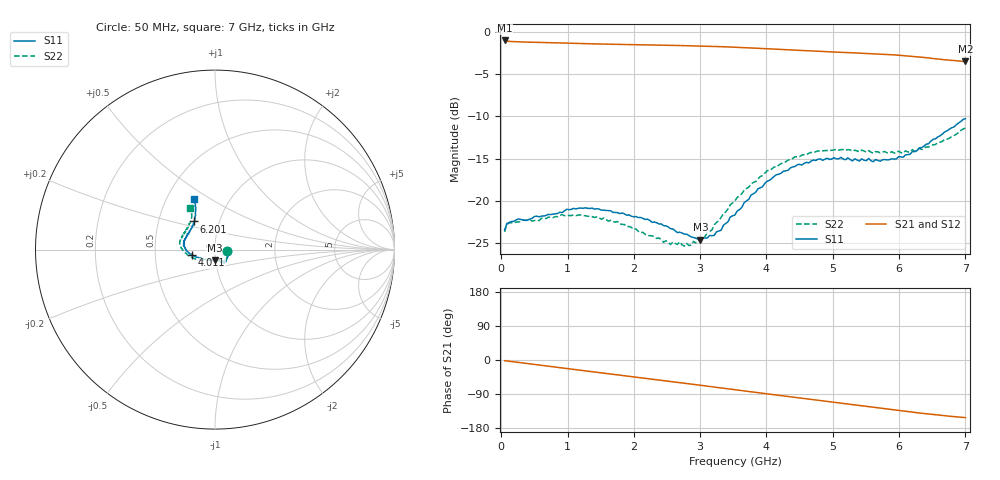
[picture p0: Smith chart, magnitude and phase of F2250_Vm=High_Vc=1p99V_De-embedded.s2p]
! Integrated Device Technology
! Corporate Headquarters
! 6024 Silver Creek Valley Road
! San Jose, CA 95138  USA
! Phone:  1-408-284-8200
! Toll Free:  1-800-223-1366
! Webpage:  http://www.idt.com/
! Timing and RF Division
! 515 Groton Road, Suite 102
! Westford, MA 01886-6024
! Device:  F2250
! Description: Voltage Variable RF Attenuator
! Frequency:  50.0 -  6000.00 MHz
! Package:  3x3 mm Thin QFN Plastic Package: 16 pin
! Ports:  2 RF, 3 DC
!  Pin  1  = GND
!  Pin  2  = NC
!  Pin  3  = RF1  = Port 1
!  Pin  4  = NC
!  Pin  5  = GND
!  Pin  6  = GND
!  Pin  7  = GND
!  Pin  8  = GND
!  Pin  9  = NC
!  Pin 10  = RF2  = Port 2
!  Pin 11  = NC
!  Pin 12  = GND
!  Pin 13  = GND
!  Pin 14  = VCNTRL
!  Pin 15  = VDD
!  Pin 16  = VMODE
! Vcntrl:  1.990 Volts
! Vmode:  +3.300 Volts
! Vdd:  +3.30  Volts
! Current:  1.319 mA
! Data:  The device was measured on a the F2250 evaluation board which has
!  individual transmission lines to the RF pins.  Data was collected
!  using a calibrated network analyzer.  The evaluation board was
!  de-embedded using a TRL calibration technique.
!  The reference plane is the edge of the package pin.
! Misc:  SN 10
!  Action Tracker AT0258
! Date Measured:  2014-11-26
! Date:  2015-10-15  MJV
! Note:
!  Integrated Device Technology supplies this data as a sample of measured
!  data at the package pin for this product.  Your particular data for this
!  product may vary.
!  Data was taken at 25 degrees C.
!  Integrated Device Technology reserves the right to change this data at anytime.
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# GHz S dB R 50
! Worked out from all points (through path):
!   201 points, 50 MHz to 7 GHz, reference 50 ohm
!   highest |S21| = -1.04 dB at 50 MHz (marker M1); lowest = -3.5 dB at 7 GHz (marker M2)
!   group delay of S21, straight-line fit = 61.1 ps
!   lowest |S11| = -24.6 dB at 3.004 GHz (marker M3), VSWR 1.13, Z = 49.5 - j5.88 ohm
!   |S11| at or under -10 dB: start of sweep to end of sweep
!   |S22| runs from -25.3 to -11.4 dB; largest |S21 - S12| = 0.0018
!   S11 on the Smith chart (normalised r, x): 50 MHz: 1.14, -0.02; 4.011 GHz: 0.77, -0.05; 6.201 GHz: 0.76, +0.25; 7 GHz: 0.68, +0.42
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0.05  -23.40 -8.4  -1.04 -1.8  -1.04 -1.8  -23.62 -9.1
0.08475  -22.63 -7.7  -1.12 -2.5  -1.12 -2.5  -22.75 -8.2
0.1195  -22.51 -8.3  -1.15 -3.3  -1.15 -3.3  -22.56 -7.8
0.91875  -21.35 -43.3  -1.34 -21.1  -1.34 -21.1  -21.60 -46.9
1.2315  -20.84 -51.0  -1.41 -27.9  -1.41 -27.9  -21.70 -57.2
1.75275  -21.36 -57.9  -1.50 -39.1  -1.50 -39.1  -22.41 -65.4
2.37825  -22.69 -58.8  -1.59 -52.7  -1.59 -52.7  -24.35 -69.9
2.552  -23.25 -63.0  -1.61 -56.6  -1.61 -56.6  -25.12 -76.5
2.691  -23.67 -69.4  -1.64 -59.7  -1.64 -59.7  -24.81 -83.3
2.7605  -23.89 -71.2  -1.65 -61.2  -1.65 -61.2  -25.32 -87.4
3.00375  -24.55 -91.7  -1.70 -66.7  -1.70 -66.7  -24.37 -108.4
3.21225  -24.03 -113.0  -1.74 -71.4  -1.74 -71.4  -22.80 -126.3
3.525  -21.62 -141.4  -1.84 -78.5  -1.84 -78.5  -19.95 -145.1
3.76825  -19.27 -156.5  -1.93 -84.0  -1.93 -84.0  -17.97 -156.7
4.0115  -17.64 -166.2  -2.03 -89.4  -2.03 -89.4  -16.41 -166.5
4.4285  -15.92 -178.6  -2.19 -98.6  -2.19 -98.6  -14.77 -179.3
4.7065  -15.15 173.9  -2.29 -104.8  -2.29 -104.8  -14.29 174.7
5.054  -15.01 165.6  -2.42 -112.4  -2.41 -112.5  -13.91 167.3
5.85325  -15.11 139.1  -2.71 -129.9  -2.71 -130.0  -14.31 148.2
6.20075  -14.15 126.8  -2.92 -137.6  -2.92 -137.7  -13.93 139.0
6.54825  -12.65 118.2  -3.19 -144.6  -3.19 -144.8  -13.32 127.6
7  -10.27 112.8  -3.52 -152.0  -3.53 -152.1  -11.36 121.2
